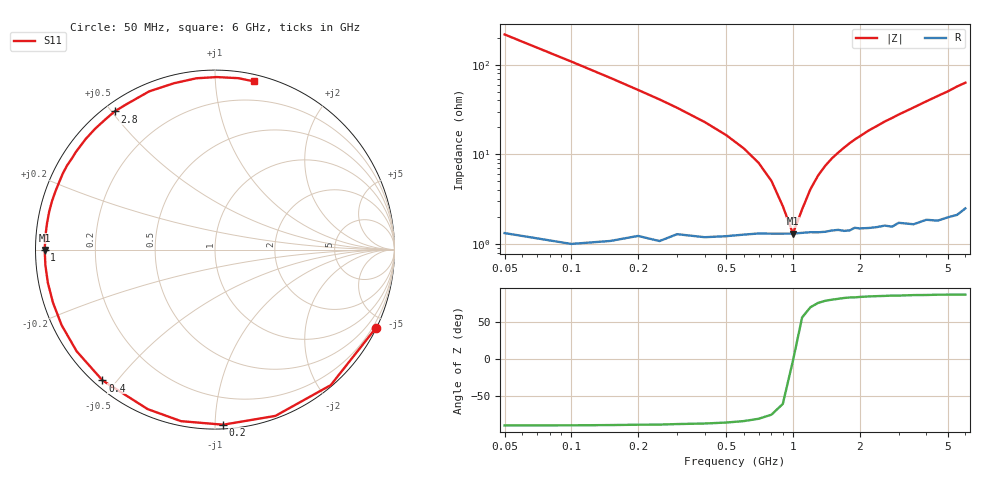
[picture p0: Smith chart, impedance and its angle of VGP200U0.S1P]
! Infineon Technologies  Discrete & RF Semiconductors
! BB 831
! Si Tuning Diode in SOD323
! VR = 0.2 V
! S-Parameters:  July  1999
# GHz  S  MA  R  50
!  f  S11
! GHz  MAG  ANG
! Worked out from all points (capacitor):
!   34 points, 50 MHz to 6 GHz, reference 50 ohm
!   read as one part to ground: C = 14.5 pF near 50 MHz
!   lowest |Z| = 1.31 ohm at 1 GHz (marker M1)
!   series resonance near 1.002 GHz, so ESL is about 1.7 nH
!   S11 on the Smith chart (normalised r, x): 50 MHz: 0.03, -4.35; 200 MHz: 0.02, -1.05; 400 MHz: 0.02, -0.46; 1 GHz: 0.03, -0.00; 2.8 GHz: 0.03, +0.51; 6 GHz: 0.05, +1.26
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0.05  0.9973 -25.9
0.1  0.993 -49.5
0.15  0.9858 -70.0
0.2  0.9767 -87.3
0.25  0.9744 -101.2
0.3  0.9647 -112.9
0.4  0.9612 -130.7
0.5  0.9566 -143.7
0.6  0.9526 -153.8
0.7  0.9499 -161.9
0.8  0.9494 -168.8
0.9  0.949 -174.7
1  0.9488 -179.9
1.1  0.9479 175.3
1.3  0.9478 167.0
1.4  0.9475 163.2
1.6  0.9461 156.5
1.9  0.9454 147.4
2.2  0.948 139.4
2.4  0.9484 134.8
2.6  0.9483 130.0
2.8  0.9514 126.0
3.5  0.9548 112.6
4  0.9546 103.9
4.5  0.9602 96.2
5  0.9613 89.4
5.5  0.9639 82.3
6  0.962 76.8
